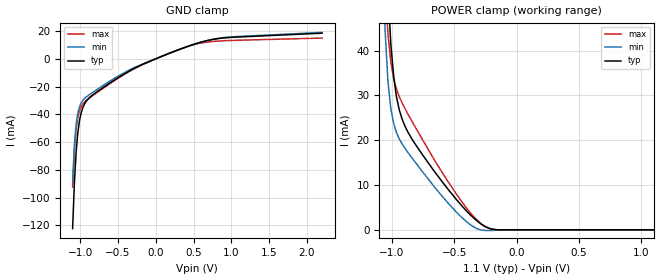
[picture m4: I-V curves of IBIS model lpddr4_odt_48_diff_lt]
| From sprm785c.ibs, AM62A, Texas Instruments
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|   Model lpddr4_odt_48_diff_lt
[Model] lpddr4_odt_48_diff_lt
Model_type Input
Polarity   Non-Inverting
Enable   Active-High
Vinl =  0.113V
Vinh =  0.253V
C_comp   2.430pF   2.307pF   2.472pF
[Model Spec]
Vinh   0.253V   0.247V   0.265V
Vinl   0.113V   0.107V   0.125V
[Temperature Range]   25.000   -40.000   -40.000
[Voltage Range]   1.100V   1.060V   1.170V
[C Comp Corner]
C_comp   2.430pF   2.307pF   2.472pF
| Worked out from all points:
|   GND clamp passes 1 mA (typ) near -0.04 V on its own axis
|   POWER clamp passes 1 mA (typ) near -0.27 V on its own axis
[GND_clamp]
|Voltage   I(typ)   I(min)   I(max)
-1.1V     -122.4mA   -88.53mA   -92.5mA
-1.077V   -89.69mA   -62.44mA   -66.08mA
-1.054V   -67.44mA   -47.31mA   -50.64mA
-1.031V   -53.13mA   -39.01mA   -42.08mA
-1.008V   -44.19mA   -34.41mA   -37.25mA
-985mV    -38.55mA   -31.66mA   -34.34mA
-940mV    -32.3mA    -28.53mA   -31.02mA
-848mV    -26.66mA   -24.76mA   -27.07mA
-229mV    -5.447mA   -5.093mA   -5.614mA
527mV     10.81mA    10.65mA    10.44mA
940mV     15.15mA    15.48mA    13.05mA
2.2V      18.41mA    18.98mA    14.89mA
[POWER_clamp]
|Voltage   I(typ)   I(min)   I(max)
-1.1V     151.8mA    106.6mA    118.3mA
-1.054V   73.1mA     44.59mA    55.65mA
-1.031V   53.42mA    33.06mA    43.77mA
-1.008V   41.48mA    27.07mA    37.45mA
-985mV    34.21mA    23.72mA    33.77mA
-963mV    29.73mA    21.7mA     31.45mA
-940mV    26.75mA    20.26mA    29.69mA
-894mV    23.12mA    18.18mA    27.05mA
-802mV    18.7mA     14.71mA    22.45mA
-367mV    3.228mA    1.063mA    3.672mA
-183mV    85.18uA    -125.3uA   64.37uA
1.1V      0A         0A         0A
